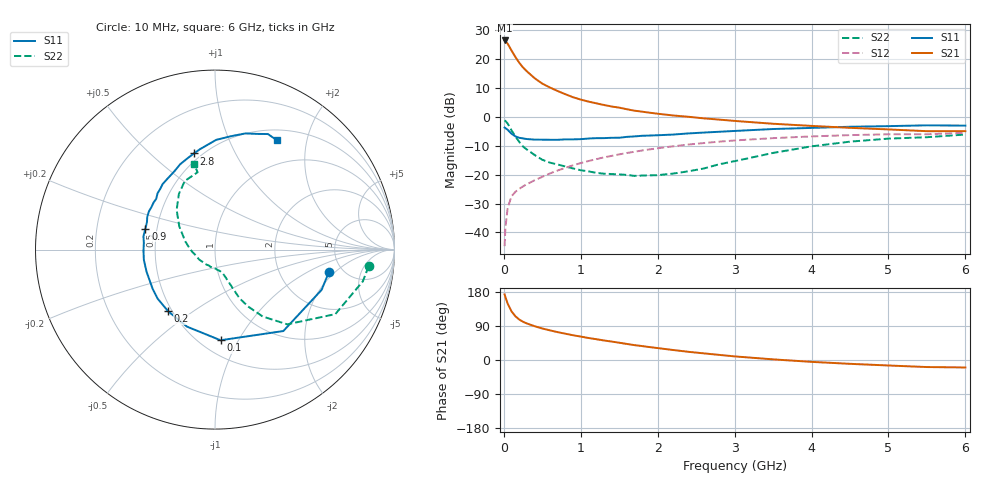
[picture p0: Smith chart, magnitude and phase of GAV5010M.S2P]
! Infineon Technologies  Discrete & RF Semiconductors
! BF775
! Si NPN RF Bipolar Junction Transistor in SOT23
! VCE = 0.5 V  IC = 10 mA
! Common Emitter S-Parameters:  May  1996
# GHz  S  MA  R  50
!  f  S11  S21  S12  S22
! GHz  MAG  ANG  MAG  ANG  MAG  ANG  MAG  ANG
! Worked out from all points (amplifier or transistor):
!   36 points, 10 MHz to 6 GHz, reference 50 ohm
!   highest |S21| = 26.3 dB at 10 MHz (marker M1)
!   |S21| within 3 dB of that: start of sweep to 89.77 MHz
!   unconditionally stable (mu >= 1): 283.4 MHz to end of sweep
!   at 250 MHz: K = 0.94, MSG = 20.5 dB, |S12| = -24.1 dB
!   at 1.4 GHz: K = 1.41, MAG = 4.7 dB, |S12| = -13.6 dB
!   at 6 GHz: K = 1.14, MAG = -2.0 dB, |S12| = -5.6 dB
!   S11 on the Smith chart (normalised r, x): 10 MHz: 3.92, -1.67; 100 MHz: 0.62, -0.85; 200 MHz: 0.48, -0.40; 900 MHz: 0.43, +0.12; 2.8 GHz: 0.46, +0.70; 6 GHz: 0.64, +1.52
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0.01  0.6472 -11.0  20.69 173.1  0.0058 81.6  0.8611 -6.2
0.02  0.6349 -20.7  20.18 166.4  0.0119 80.7  0.8426 -12.1
0.05  0.5923 -50.0  18.16 148.8  0.0266 67.2  0.7607 -28.2
0.1  0.506 -86.5  13.86 128.2  0.0422 55.2  0.5789 -46.0
0.15  0.4567 -110.0  10.75 115.4  0.0503 50.9  0.458 -54.5
0.2  0.4316 -127.2  8.546 106.8  0.0567 49.9  0.3668 -59.8
0.25  0.4204 -139.5  7.056 100.8  0.0625 50.0  0.3043 -63.2
0.3  0.4106 -147.7  6.055 96.4  0.0682 51.5  0.2703 -64.2
0.4  0.4008 -162.0  4.614 89.2  0.0797 53.5  0.2178 -66.1
0.5  0.4005 -171.7  3.717 83.1  0.0914 55.5  0.1801 -68.1
0.6  0.3986 -178.7  3.183 78.2  0.1045 56.5  0.1605 -69.5
0.7  0.3982 174.5  2.767 73.5  0.1177 57.1  0.1491 -70.6
0.9  0.4052 163.3  2.164 65.3  0.1445 56.9  0.1274 -75.2
1.1  0.419 154.3  1.82 58.1  0.1712 55.7  0.1135 -83.5
1.3  0.4258 146.5  1.592 51.6  0.1978 53.8  0.1036 -91.3
1.7  0.4562 131.8  1.267 39.2  0.2481 49.3  0.0949 -111.8
2.2  0.4908 117.6  1.048 26.4  0.3077 42.4  0.1039 -147.3
2.8  0.5485 102.4  0.889 13.5  0.3703 33.5  0.1506 172.6
3.5  0.6114 89.4  0.754 1.7  0.4257 22.9  0.2365 147.2
4.5  0.6693 75.3  0.641 -10.1  0.4798 9.1  0.3701 122.9
5.5  0.7081 65.4  0.561 -18.6  0.4965 -3.5  0.4416 102.7
6  0.7 60.4  0.562 -19.7  0.5262 -7.1  0.4916 103.8
